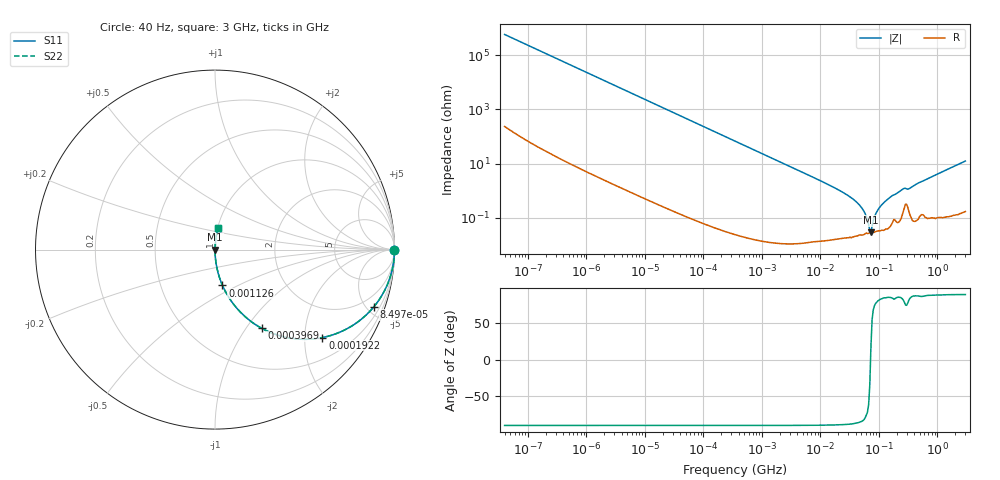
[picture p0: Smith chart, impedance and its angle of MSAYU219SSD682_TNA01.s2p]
! MSAYU219SSD682_TNA01  S-PARAMETER MODEL  ( General Type )
! Model Generated by TAIYO YUDEN Corporation (http://www.ty-top.com)
! Version 2.0
! TAIYO YUDEN Control No. 031016
! Copyright(c) 2003 TAIYO YUDEN CO.,LTD. All Rights Reserved.
! Product Description (link to TY-COMPAS)
! https://ds.yuden.co.jp/TYCOMPAS/or/detail?pn=MSAYU219SSD682KTNA01&u=M
! Products Name : Multilayer Ceramic Capacitors
! Characteristics :
!  Capacitance : 6800 pF , Rated Voltage : 50V
!  Case Size : 2.0 x 1.25 / 0.079 x 0.049 [mm/inch] , Thickness : 0.85 / 0.033 [mm/inch]
!  (Conditions: Temperature = 25 degC , DC Bias Current/Voltage = 0A / 0V)
! External Node Assignments :
!  1  o---| |---o  2
! GND o---------o GND
! Frequency Range : 40Hz  -  3GHz  [ 401 STEP ]
# MHz S RI R 50
! Freq[MHz].  S11 Real  S11 Imag  S21 Real  S21 Imag  S12 Real  S12 Imag  S22 Real  S22 Imag
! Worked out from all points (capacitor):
!   401 points, 40 Hz to 3 GHz, reference 50 ohm
!   read as one part in series: C = 6.78 nF near 44 Hz
!   lowest |Z| = 28.8 mohm at 72.9 MHz (marker M1)
!   series resonance near 71.88 MHz, so ESL is about 720 pH
!   S11 on the Smith chart (normalised r, x): 40 Hz: open; 84.97 kHz: 1.00, -5.52; 192.2 kHz: 1.00, -2.44; 396.9 kHz: 1.00, -1.18; 1.126 MHz: 1.00, -0.42; 3 GHz: 1.00, +0.25
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4e-05  1 -0.00017  9.7e-08 0.00017  9.7e-08 0.00017  1 -0.00017
0.000834  1 -0.00355  1.34e-05 0.00355  1.34e-05 0.00355  1 -0.00355
0.017386  0.9945 -0.0737  0.00547 0.0737  0.00547 0.0737  0.9945 -0.0737
0.084972  0.8841 -0.32  0.1159 0.32  0.1159 0.32  0.8841 -0.32
0.192155  0.5987 -0.49  0.4013 0.49  0.4013 0.49  0.5987 -0.49
0.362475  0.2955 -0.4561  0.7045 0.4561  0.7045 0.4561  0.2955 -0.4561
0.396875  0.2592 -0.438  0.7408 0.438  0.7408 0.438  0.2592 -0.438
1.125822  0.0417 -0.1997  0.9583 0.1997  0.9583 0.1997  0.0417 -0.1997
7.222098  0.00116 -0.0321  0.9988 0.0321  0.9988 0.0321  0.00116 -0.0321
21.43715  0.000265 -0.00994  0.9997 0.00994  0.9997 0.00994  0.000265 -0.00994
38.64618  0.00022 -0.00428  0.9998 0.00428  0.9998 0.00428  0.00022 -0.00428
53.07868  0.000232 -0.00198  0.9998 0.00198  0.9998 0.00198  0.000232 -0.00198
58.11596  0.000255 -0.00137  0.9997 0.00137  0.9997 0.00137  0.000255 -0.00137
66.58224  0.000263 -0.000487  0.9997 0.000487  0.9997 0.000487  0.000263 -0.000487
72.90103  0.000275 8.61e-05  0.9997 -8.61e-05  0.9997 -8.61e-05  0.000275 8.61e-05
76.28187  0.000279 0.000392  0.9997 -0.000392  0.9997 -0.000392  0.000279 0.000392
87.39454  0.000303 0.00129  0.9997 -0.00129  0.9997 -0.00129  0.000303 0.00129
95.68847  0.000321 0.00189  0.9997 -0.00189  0.9997 -0.00189  0.000321 0.00189
150.5692  0.000462 0.00534  0.9995 -0.00534  0.9995 -0.00534  0.000462 0.00534
259.4108  0.00176 0.0114  0.9982 -0.0114  0.9982 -0.0114  0.00176 0.0114
340.4975  0.00137 0.0123  0.9986 -0.0123  0.9986 -0.0123  0.00137 0.0123
3000  0.0166 0.1211  0.9834 -0.1211  0.9834 -0.1211  0.0166 0.1211
